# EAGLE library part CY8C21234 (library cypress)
PSoC® Programmable System-on-Chip? M8C Processor Speeds to 24 MHz Source: http://www.cypress.com .. 38-12025_0P_V.pdf
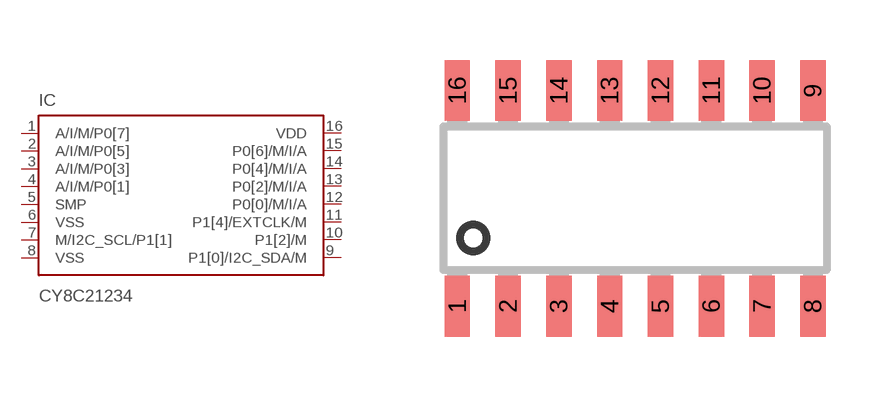
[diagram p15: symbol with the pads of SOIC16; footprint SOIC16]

Designator prefix IC

## CY8C21234 (MPN: CY8C21234-24SXI; OC_FARNELL: 1321728; OC_NEWARK: 19M7160)  [SOIC16]
1  A/I/M/P0[7]
2  A/I/M/P0[5]
3  A/I/M/P0[3]
4  A/I/M/P0[1]
5  SMP  pwr
6  VSS  pwr
7  M/I2C_SCL/P1[1]
8  VSS  pwr
9  P1[0]/I2C_SDA/M
10  P1[2]/M
11  P1[4]/EXTCLK/M
12  P0[0]/M/I/A
13  P0[2]/M/I/A
14  P0[4]/M/I/A
15  P0[6]/M/I/A
16  VDD  pwr

## Footprint SOIC16 (pad centres in mm)
SMALL OUTLINE INTEGRATED CIRCUIT 16-Pin (150-Mil) SOIC Source: http://www.cypress.com .. 38-12025_0P_V.pdf
smd 0.635 x 1.524: 1 -4.445,-2.695; 2 -3.175,-2.695; 3 -1.905,-2.695; 4 -0.635,-2.695; 5 0.635,-2.695; 6 1.905,-2.695; 7 3.175,-2.695; 8 4.445,-2.695; 9 4.445,2.695; 10 3.175,2.695; 11 1.905,2.695; 12 0.635,2.695; 13 -0.635,2.695; 14 -1.905,2.695; 15 -3.175,2.695; 16 -4.445,2.695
